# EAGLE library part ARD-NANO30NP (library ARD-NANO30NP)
Development Boards & Kits - AVR Arduino Nano 3.1 W/ATMEGA328 NO-PIN Source: Datasheet
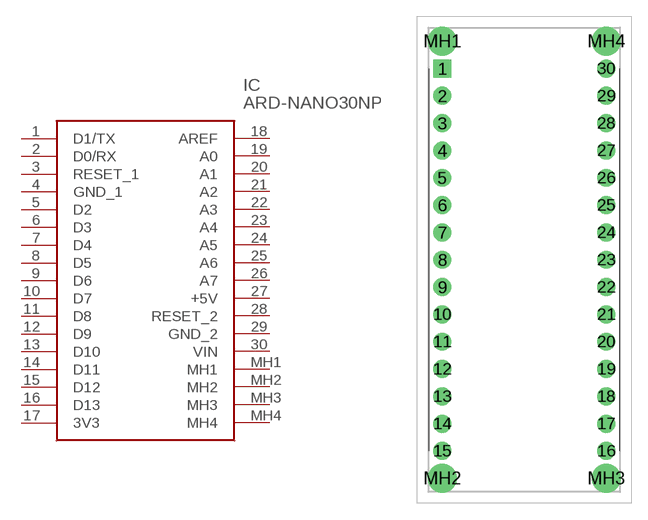
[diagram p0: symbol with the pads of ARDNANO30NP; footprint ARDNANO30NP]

Designator prefix IC

## ARD-NANO30NP (Description: Development Boards & Kits - AVR Arduino Nano 3.1 W/ATMEGA328 NO-PIN; Height: 5mm; Manufacturer_Name: Gravitech; Manufacturer_Part_Number: ARD-NANO30NP; Mouser_Part_Number: 992-ARD-NANO30NP; Mouser_Price-Stock: https://www.mouser.com/Search/Refine.aspx?Keyword=992-ARD-NANO30NP)  [ARDNANO30NP]
1  D1/TX
2  D0/RX
3  RESET_1
4  GND_1
5  D2
6  D3
7  D4
8  D5
9  D6
10  D7
11  D8
12  D9
13  D10
14  D11
15  D12
16  D13
17  3V3
18  AREF
19  A0
20  A1
21  A2
22  A3
23  A4
24  A5
25  A6
26  A7
27  +5V
28  RESET_2
29  GND_2
30  VIN
MH1  MH1
MH2  MH2
MH3  MH3
MH4  MH4

## Footprint ARDNANO30NP (pad centres in mm)
ARD-NANO30NP-4
drill 1.11 pad 1.665 square: 1 0,0
drill 1.11 pad 1.665: 2 0,-2.54; 3 0,-5.08; 4 0,-7.62; 5 0,-10.16; 6 0,-12.7; 7 0,-15.24; 8 0,-17.78; 9 0,-20.32; 10 0,-22.86; 11 0,-25.4; 12 0,-27.94; 13 0,-30.48; 14 0,-33.02; 15 0,-35.56; 16 15.24,-35.56; 17 15.24,-33.02; 18 15.24,-30.48; 19 15.24,-27.94; 20 15.24,-25.4; 21 15.24,-22.86; 22 15.24,-20.32; 23 15.24,-17.78; 24 15.24,-15.24; 25 15.24,-12.7; 26 15.24,-10.16; 27 15.24,-7.62; 28 15.24,-5.08; 29 15.24,-2.54; 30 15.24,0
drill 1.778 pad 2.667: MH1 0,2.54; MH2 0,-38.1; MH3 15.24,-38.1; MH4 15.24,2.54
